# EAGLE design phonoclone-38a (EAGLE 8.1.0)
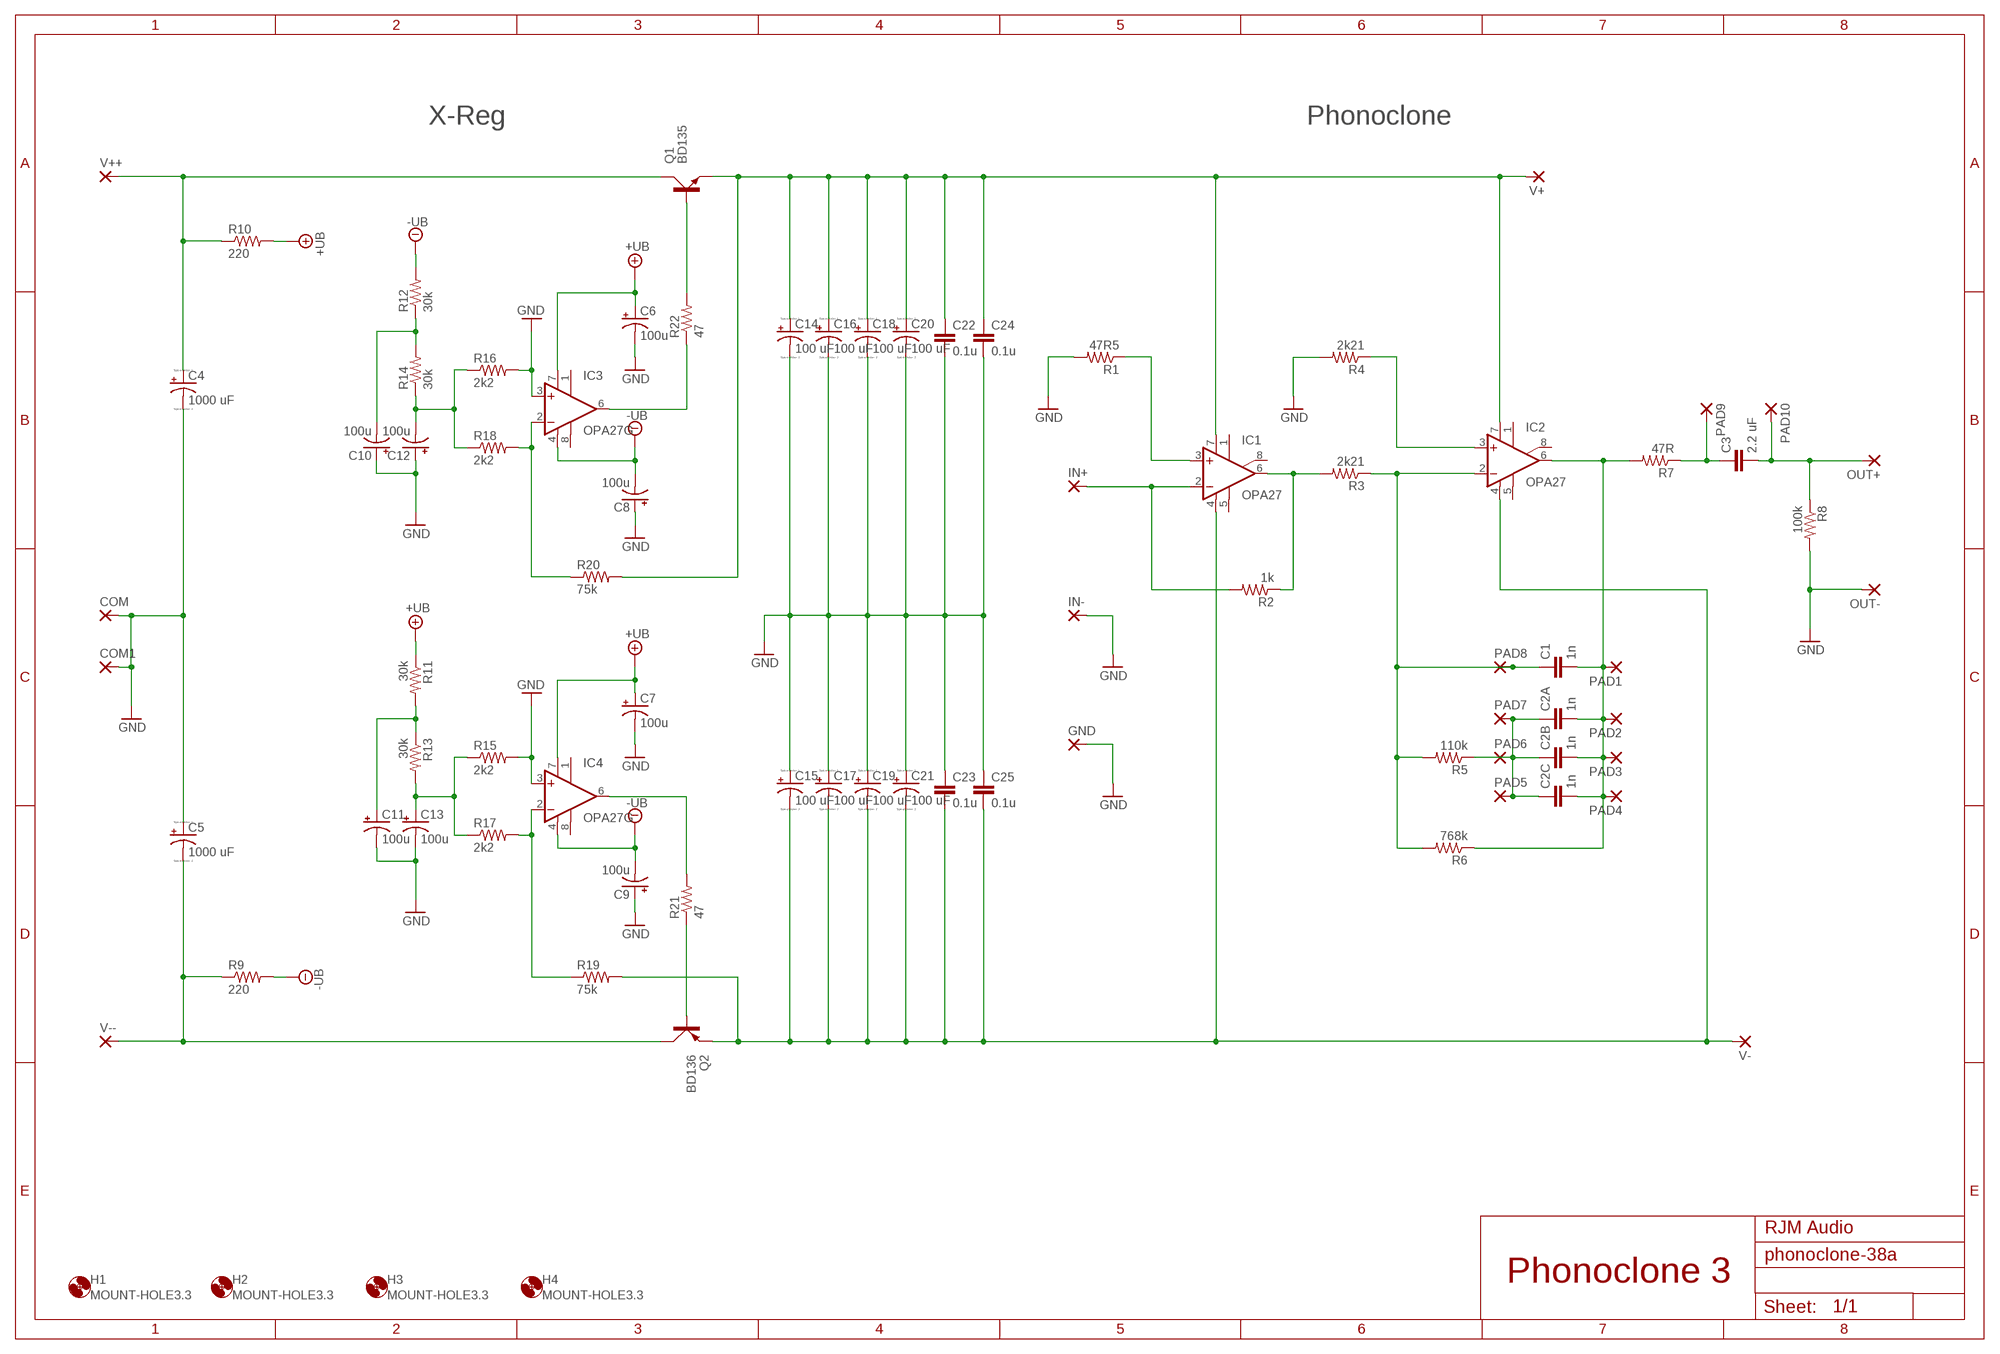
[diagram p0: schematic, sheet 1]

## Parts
C1  1n  C-EU050-045X075  [C050-045X075]
C2A  1n  C-EU050-045X075  [C050-045X075]
C2B  1n  C-EU050-045X075  [C050-045X075]
C2C  1n  C-EU050-045X075  [C050-045X075]
C3  2.2 uF  C-EU375-155X418  [C375-155X418]
C4  1000 uF  CPOL-USE5-10.5  [E5-10,5]
C5  1000 uF  CPOL-USE5-10.5  [E5-10,5]
C6  100u  CPOL-USE2.5-6  [E2,5-6]
C7  100u  CPOL-USE2.5-6  [E2,5-6]
C8  100u  CPOL-USE2.5-6  [E2,5-6]
C9  100u  CPOL-USE2.5-6  [E2,5-6]
C10  100u  CPOL-USE2.5-6  [E2,5-6]
C11  100u  CPOL-USE2.5-6  [E2,5-6]
C12  100u  CPOL-USE2.5-6  [E2,5-6]
C13  100u  CPOL-USE2.5-6  [E2,5-6]
C14  100 uF  CPOL-USE2.5-6  [E2,5-6]
C15  100 uF  CPOL-USE2.5-6  [E2,5-6]
C16  100 uF  CPOL-USE2.5-6  [E2,5-6]
C17  100 uF  CPOL-USE2.5-6  [E2,5-6]
C18  100 uF  CPOL-USE2.5-6  [E2,5-6]
C19  100 uF  CPOL-USE2.5-6  [E2,5-6]
C20  100 uF  CPOL-USE2.5-6  [E2,5-6]
C21  100 uF  CPOL-USE2.5-6  [E2,5-6]
C22  0.1u  C-EU050-024X044  [C050-024X044]
C23  0.1u  C-EU050-024X044  [C050-024X044]
C24  0.1u  C-EU050-024X044  [C050-024X044]
C25  0.1u  C-EU050-024X044  [C050-024X044]
COM  3,17/1,3  [3,17/1,3]
COM1  3,17/1,3  [3,17/1,3]
GND  3,17/1,3  [3,17/1,3]
H1  MOUNT-HOLE3.3  [3,3]
H2  MOUNT-HOLE3.3  [3,3]
H3  MOUNT-HOLE3.3  [3,3]
H4  MOUNT-HOLE3.3  [3,3]
IC1  OPA27  OPA124P  [DIL08]
IC2  OPA27  OPA124P  [DIL08]
IC3  OPA27G  OPA134P  [DIL08]
IC4  OPA27G  OPA134P  [DIL08]
IN+  3,17/1,3  [3,17/1,3]
IN-  3,17/1,3  [3,17/1,3]
OUT+  3,17/1,3  [3,17/1,3]
OUT-  3,17/1,3  [3,17/1,3]
PAD1  2,15/1,0  [2,15/1,0]
PAD2  2,15/1,0  [2,15/1,0]
PAD3  2,15/1,0  [2,15/1,0]
PAD4  2,15/1,0  [2,15/1,0]
PAD5  2,15/1,0  [2,15/1,0]
PAD6  2,15/1,0  [2,15/1,0]
PAD7  2,15/1,0  [2,15/1,0]
PAD8  2,15/1,0  [2,15/1,0]
PAD9  3,17/1,3  [3,17/1,3]
PAD10  3,17/1,3  [3,17/1,3]
Q1  BD135  BD139  [TO126AV]
Q2  BD136  BD140  [TO126AV]
R1  47R5  R-US_0207/10  [0207/10]
R2  1k  R-US_0207/10  [0207/10]
R3  2k21  R-US_0207/10  [0207/10]
R4  2k21  R-US_0207/10  [0207/10]
R5  110k  R-US_0207/10  [0207/10]
R6  768k  R-US_0207/10  [0207/10]
R7  47R  R-US_0207/10  [0207/10]
R8  100k  R-US_0207/10  [0207/10]
R9  220  R-US_0207/10  [0207/10]
R10  220  R-US_0207/10  [0207/10]
R11  30k  R-US_0207/10  [0207/10]
R12  30k  R-US_0207/10  [0207/10]
R13  30k  R-US_0207/10  [0207/10]
R14  30k  R-US_0207/10  [0207/10]
R15  2k2  R-US_0207/10  [0207/10]
R16  2k2  R-US_0207/10  [0207/10]
R17  2k2  R-US_0207/10  [0207/10]
R18  2k2  R-US_0207/10  [0207/10]
R19  75k  R-US_0207/10  [0207/10]
R20  75k  R-US_0207/10  [0207/10]
R21  47  R-US_0207/10  [0207/10]
R22  47  R-US_0207/10  [0207/10]
V+  2,15/1,0  [2,15/1,0]
V++  3,17/1,3  [3,17/1,3]
V-  2,15/1,0  [2,15/1,0]
V--  3,17/1,3  [3,17/1,3]

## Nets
+UB: C6.+ C7.+ IC3.7(V+) IC4.7(V+) R10.2 R11.1
-UB: C8.- C9.- IC3.4(V-) IC4.4(V-) R9.2 R12.2
GND: C4.- C5.+ C6.- C7.- C8.+ C9.+ C10.+ C11.- C12.+ C13.- C14.- C15.+ C16.- C17.+ C18.- C19.+ C20.- C21.+ C22.2 C23.1 C24.2 C25.1 COM1.1(P) COM.1(P) GND.1(P) IC3.3(+IN) IC4.3(+IN) IN-.1(P) OUT-.1(P) R1.2 R4.2 R8.2 R15.2 R16.2
N$1: IC1.6(OUT) R2.1 R3.2
N$2: IC1.3(+IN) R1.1
N$3: IC2.3(+IN) R4.1
N$4: IC3.6(OUT) R22.1
N$5: C2A.1 C2B.1 C2C.1 PAD5.1(P) PAD6.1(P) PAD7.1(P) R5.1
N$6: C1.1 IC2.2(-IN) PAD8.1(P) R3.1 R5.2 R6.2
N$7: Q1.B R22.2
N$8: C11.+ R11.2 R13.1
N$9: IC4.2(-IN) R17.2 R19.1
N$10: Q2.B R21.1
N$11: IC4.6(OUT) R21.2
N$13: IC3.2(-IN) R18.2 R20.1
N$14: C10.- R12.1 R14.2
N$16: C3.1 PAD9.1(P) R7.1
NINV: IC1.2(-IN) IN+.1(P) R2.2
OUT: C1.2 C2A.2 C2B.2 C2C.2 IC2.6(OUT) PAD1.1(P) PAD2.1(P) PAD3.1(P) PAD4.1(P) R6.1 R7.2
OUT+: C3.2 OUT+.1(P) PAD10.1(P) R8.1
V+: C14.+ C16.+ C18.+ C20.+ C22.1 C24.1 IC1.7(V+) IC2.7(V+) Q1.E R20.2 V+.1(P)
V++: C4.+ Q1.C R10.1 V++.1(P)
V-: C15.- C17.- C19.- C21.- C23.2 C25.2 IC1.4(V-) IC2.4(V-) Q2.E R19.2 V-.1(P)
V--: C5.- Q2.C R9.1 V--.1(P)
VREF+: C13.+ R13.2 R15.1 R17.1
VREF-: C12.- R14.1 R16.1 R18.1
Unconnected: IC1.1(TRIM1) IC1.5(TRIM2) IC1.8(SUBS) IC2.1(TRIM1) IC2.5(TRIM2) IC2.8(SUBS) IC3.1(TRIM1) IC3.8(TRIM2) IC4.1(TRIM1) IC4.8(TRIM2)

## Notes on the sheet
- X-Reg | Phonoclone
- RJM Audio
- Phonoclone 3

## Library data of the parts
C1 C2A C2B C2C C3 = resistor:C-EU: CAPACITOR, European symbol
C4 C5 C14-C21 = resistor:CPOL-US: POLARIZED CAPACITOR, American symbol
C6-C13 = rcl:CPOL-US: POLARIZED CAPACITOR, American symbol
C22-C25 = rcl:C-EU: CAPACITOR, European symbol
COM COM1 GND IN+ IN- OUT+ OUT- PAD9 PAD10 V++ V-- = wirepad:3,17/1,3: THROUGH-HOLE PAD
H1-H4 = holes:MOUNT-HOLE: MOUNTING HOLE with drill center marker
IC1 IC2 = burr-brown:OPA124: Difet Operational Amplifier Low Noise, Precision; OC_FARNELL: unknown; OC_NEWARK: unknown
IC3 IC4 = burr-brown:OPA134: Operational Amplifiers SoundPlus(TM) High Performance Audio; MF: TEXAS INSTRUMENTS; MPN: OPA134PA; OC_FARNELL: 1335032; OC_NEWARK: 75C4599
PAD1-PAD8 V+ V- = wirepad:2,15/1,0: THROUGH-HOLE PAD
Q1 = transistor-power:BD139: NPN TRANSISTOR
Q2 = transistor-power:BD140: PNP TRANSISTOR
R1-R8 = resistor:R-US_: RESISTOR, American symbol
R9-R22 = rcl:R-US_: RESISTOR, American symbol

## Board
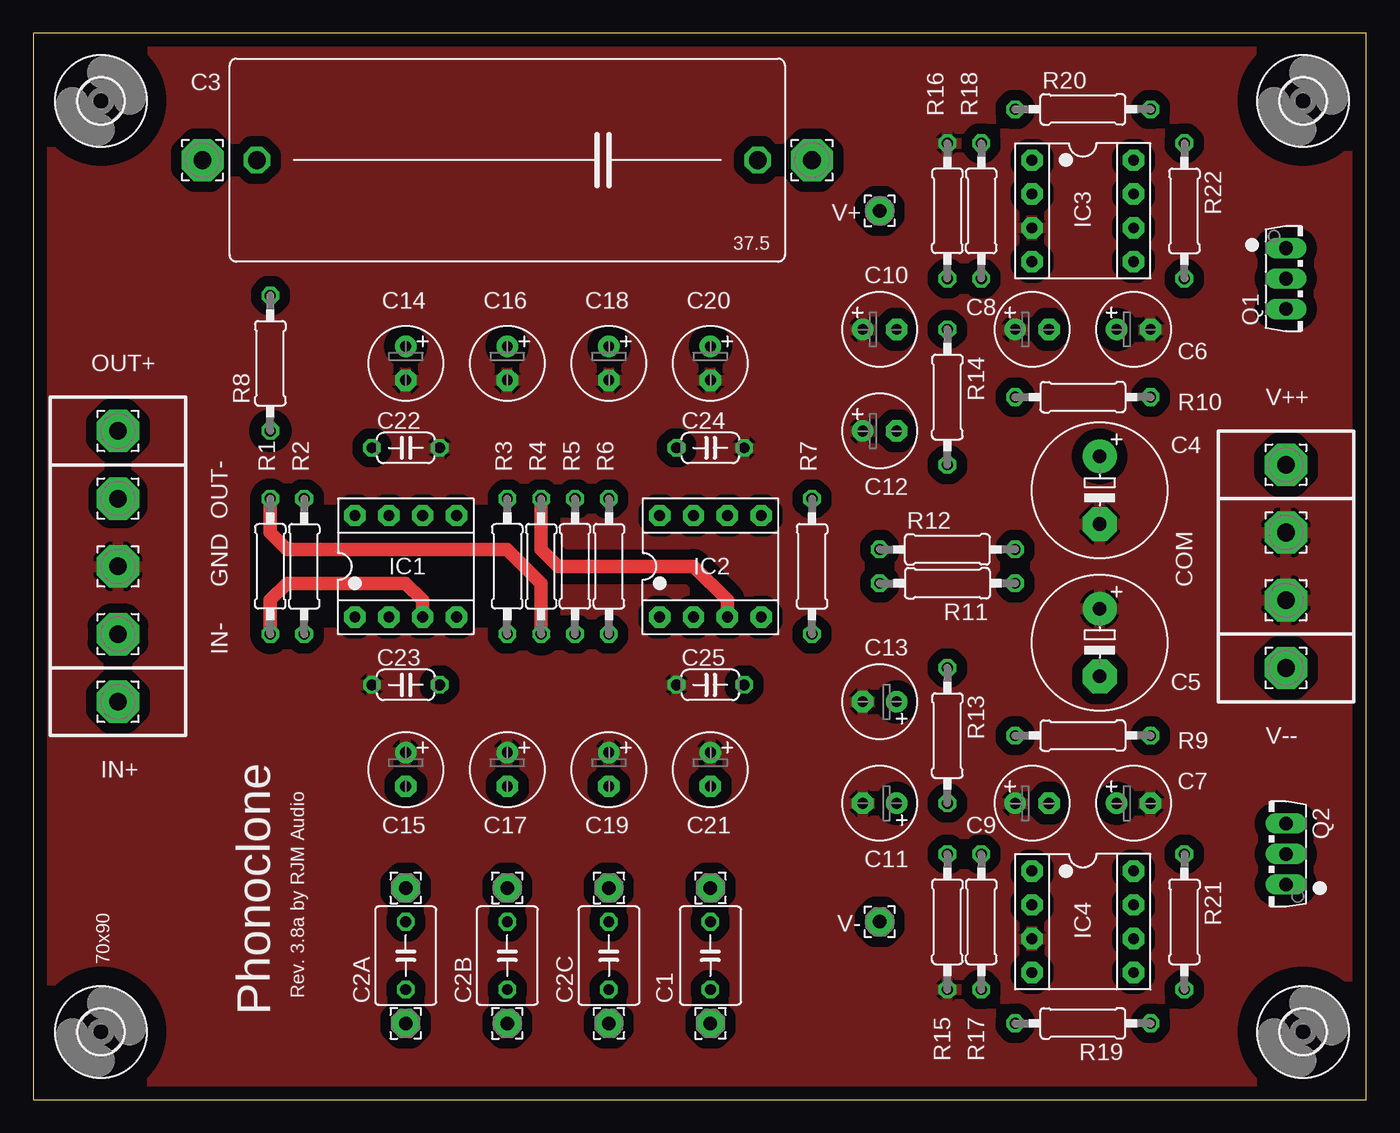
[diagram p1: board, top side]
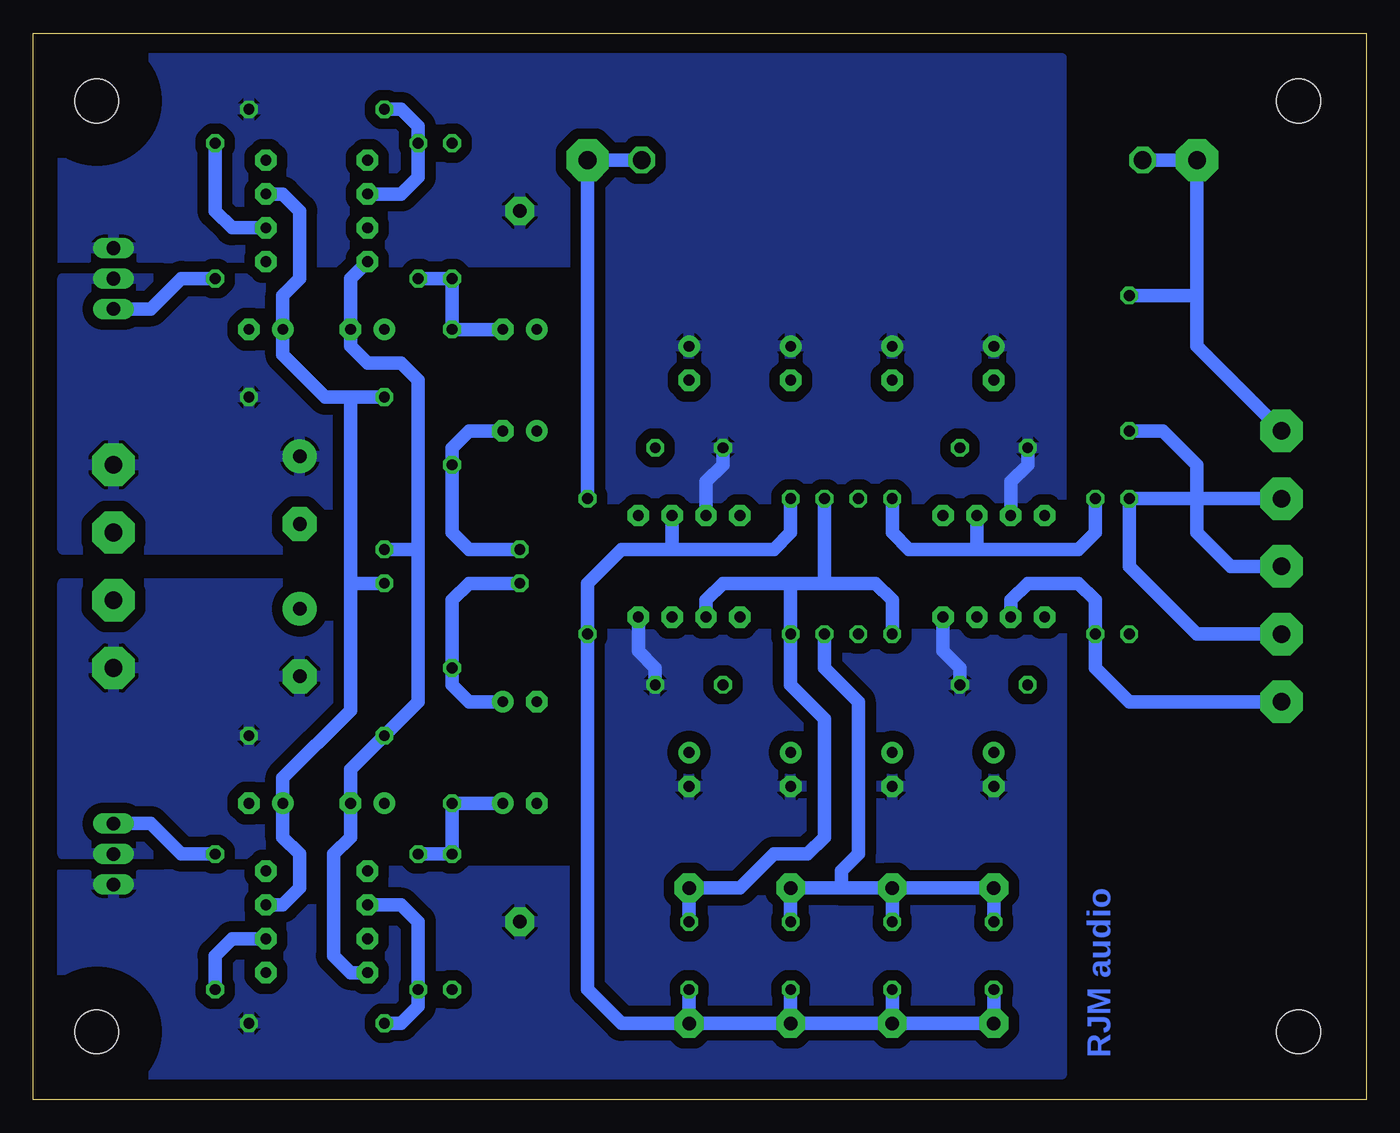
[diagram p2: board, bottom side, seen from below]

Size 100 x 80 mm. Coordinates in mm from the lower left corner, seen from the top.
Outline: 0,0 100,0 100,80 0,80 0,0
Copper layers (1*16): Top 0.035mm / dielectric 1.5mm / Bottom 0.035mm
Design rules "default": minimum track width 10mil, minimum drill 24mil, track to track 8mil, track to pad 8mil, pad to pad 8mil, via to via 8mil, smd to smd 8mil, copper to edge 40mil, drill to drill 8mil, minimum pad ring 10mil, minimum via ring 8mil, stop-mask expansion 4mil, vias tented up to drill 0mil, thermal gap 10mil
tRestrict: area 17.1,49.5 to 18.4,50.8; area 37.5,34.3 to 38.7,35.6; area 18.4,36.2 to 38.7,43.8; 17 lines

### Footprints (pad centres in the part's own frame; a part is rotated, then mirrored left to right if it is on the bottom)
C050-045X075 = drill 0.813 octagon: 1 -2.54,0; 2 2.54,0
C375-155X418 = drill 1.321 octagon: 1 -18.796,0; 2 18.796,0
E5-10,5 = drill 1.016 pad 2.54: + -2.54,0 | drill 1.016 pad 2.54 octagon: - 2.54,0
E2,5-6 = drill 0.813 pad 1.6: + -1.27,0 | drill 0.813 pad 1.6 octagon: - 1.27,0
C050-024X044 = drill 0.813 octagon: 1 -2.54,0; 2 2.54,0
3,17/1,3 = drill 1.321 pad 3.175 octagon: 1 0,0
3,3 = hole 3.3: 0,0
DIL08 = drill 0.813 pad 1.6 octagon: 1 -3.81,-3.81; 2 -1.27,-3.81; 3 1.27,-3.81; 4 3.81,-3.81; 5 3.81,3.81; 6 1.27,3.81; 7 -1.27,3.81; 8 -3.81,3.81
2,15/1,0 = drill 1.016 pad 2.159 octagon: 1 0,0
TO126AV = drill 1.016 long: B 2.286,-1.27; C 0,-1.27; E -2.286,-1.27
0207/10 = drill 0.813 octagon: 1 -5.08,0; 2 5.08,0

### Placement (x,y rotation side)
C1  50.8,10.79 270 top
C2A  27.94,10.79 270 top
C2B  35.56,10.79 270 top
C2C  43.18,10.79 270 top
C3  35.56,70.48 180 top
C4  80.01,45.72 270 top
C5  80.01,34.29 270 top
C6  82.55,57.79 0 top
C7  82.55,22.22 0 top
C8  74.93,57.79 0 top
C9  74.93,22.22 0 top
C10  63.5,50.16 0 top
C11  63.5,29.84 180 top
C12  63.5,57.79 0 top
C13  63.5,22.22 180 top
C14  27.94,55.25 270 top
C15  27.94,24.76 270 top
C16  35.56,55.25 270 top
C17  35.56,24.76 270 top
C18  43.18,55.25 270 top
C19  43.18,24.76 270 top
C20  50.8,55.25 270 top
C21  50.8,24.76 270 top
C22  27.94,48.9 0 top
C23  27.94,31.11 0 top
C24  50.8,48.9 0 top
C25  50.8,31.11 0 top
COM  93.98,37.47 0 top
COM1  93.98,42.55 0 top
GND  6.35,40.01 0 top
H1  5.08,74.93 0 top
H2  95.25,74.93 0 top
H3  5.08,5.08 0 top
H4  95.25,5.08 0 top
IC1  27.94,40.01 0 top
IC2  50.8,40.01 0 top
IC3  78.74,66.67 270 top
IC4  78.74,13.34 270 top
IN+  6.35,29.84 0 top
IN-  6.35,34.93 0 top
OUT+  6.35,50.16 0 top
OUT-  6.35,45.09 0 top
PAD1  27.94,5.71 0 top
PAD2  35.56,5.71 0 top
PAD3  43.18,5.71 0 top
PAD4  50.8,5.71 0 top
PAD5  35.56,15.88 0 top
PAD6  43.18,15.88 0 top
PAD7  27.94,15.88 0 top
PAD8  50.8,15.88 0 top
PAD9  58.42,70.48 0 top
PAD10  12.7,70.48 0 top
Q1  95.25,61.59 270 top
Q2  92.71,18.41 90 top
R1  17.78,40.01 90 top
R2  20.32,40.01 270 top
R3  35.56,40.01 90 top
R4  38.1,40.01 270 top
R5  40.64,40.01 90 top
R6  43.18,40.01 270 top
R7  58.42,40.01 270 top
R8  17.78,55.25 270 top
R9  78.74,27.3 180 top
R10  78.74,52.71 180 top
R11  68.58,38.73 180 top
R12  68.58,41.27 0 top
R13  68.58,27.3 270 top
R14  68.58,52.71 270 top
R15  68.58,13.34 270 top
R16  68.58,66.67 90 top
R17  71.12,13.34 270 top
R18  71.12,66.67 90 top
R19  78.74,5.71 0 top
R20  78.74,74.3 0 top
R21  86.36,13.34 270 top
R22  86.36,66.67 270 top
V+  63.5,66.67 0 top
V++  93.98,47.62 0 top
V-  63.5,13.34 180 top
V--  93.98,32.39 0 top

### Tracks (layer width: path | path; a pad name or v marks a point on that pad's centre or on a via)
+UB
  Bottom 1.016: IC3.7 81.28,67.94 80.01,66.67 80.01,61.59 81.28,60.33 C6.+ 81.28,55.88 78.11,52.71 76.2,52.71 | 76.2,38.73 76.2,52.71 | 76.2,52.71 R10.2 | R11.1 76.2,38.73 | 76.2,38.73 76.2,29.21 81.28,24.13 C7.+ 81.28,19.68 80.01,18.41 80.01,15.88 81.28,14.61 IC4.7
-UB
  Bottom 1.016: IC3.4 76.2,61.59 C8.- 76.2,56.52 74.93,55.25 72.39,55.25 71.12,53.98 71.12,41.27 | IC4.4 76.2,9.53 77.47,10.79 77.47,18.41 76.2,19.68 C9.- 76.2,24.76 R9.2 71.12,29.84 71.12,41.27 | R12.2 71.12,41.27
GND
  Top 1.016: R1.2 17.78,42.55 19.05,41.27 35.56,41.27 38.1,38.73 R4.2
  Bottom 1.016: 12.7,45.09 12.7,47.62 15.24,50.16 R8.2 | IN-.1 12.7,34.93 17.78,40.01 R1.2 12.7,45.09 | 12.7,45.09 OUT-.1 | GND.1 10.16,40.01 12.7,42.55 12.7,45.09
  pour Top (isolate 0.813): -1.27,81.28 101.6,81.28 101.6,-1.91 -1.27,-1.91
N$1
  Bottom 1.016: R2.1 20.32,42.55 21.59,41.27 29.21,41.27 | R3.2 35.56,42.55 34.29,41.27 29.21,41.27 | 29.21,41.27 IC1.6
N$2
  Top 1.016: IC1.3 29.21,37.47 27.94,38.73 19.05,38.73 17.78,37.47 R1.1
N$3
  Top 1.016: R4.1 38.1,41.27 39.37,40.01 49.53,40.01 52.07,37.47 IC2.3
N$4
  Bottom 1.016: IC3.6 85.09,65.41 86.36,66.67 R22.1
N$5
  Bottom 1.016: C2C.1 PAD6.1 39.37,15.88 | C2B.1 PAD5.1 | C2A.1 PAD7.1 PAD5.1 | R5.1 40.64,32.39 38.1,29.84 38.1,18.41 39.37,17.14 39.37,15.88 | 39.37,15.88 PAD5.1
N$6
  Bottom 1.016: C1.1 PAD8.1 46.99,15.88 44.45,18.41 41.91,18.41 40.64,19.68 40.64,28.57 43.18,31.11 R6.2 43.18,38.73 | R3.1 35.56,37.47 36.83,38.73 40.64,38.73 | IC2.2 49.53,37.47 48.26,38.73 43.18,38.73 | 43.18,38.73 40.64,38.73 | 40.64,38.73 R5.2
N$7
  Bottom 1.016: Q1.B 91.19,59.31 88.9,61.59 R22.2
N$8
  Bottom 1.016: R11.2 67.31,38.73 68.58,37.47 R13.1 68.58,31.11 67.31,29.84 C11.+
N$9
  Bottom 1.016: IC4.2 72.39,14.61 71.12,13.34 R17.2 71.12,6.99 72.39,5.71 R19.1
N$10
  Bottom 1.016: Q2.B 91.19,20.7 88.9,18.41 R21.1
N$11
  Bottom 1.016: IC4.6 85.09,12.06 86.36,10.79 R21.2
N$13
  Bottom 1.016: IC3.2 72.39,67.94 71.12,69.21 R18.2 71.12,73.02 72.39,74.3 R20.1
N$14
  Bottom 1.016: C10.- 67.31,50.16 68.58,48.9 R14.2 68.58,42.55 67.31,41.27 R12.1
N$16
  Bottom 1.016: R7.1 PAD9.1 C3.1
NINV
  Bottom 1.016: IC1.2 26.67,37.47 25.4,38.73 21.59,38.73 20.32,37.47 R2.2 20.32,32.39 17.78,29.84 IN+.1
OUT
  Bottom 1.016: C2C.2 PAD3.1 | C2B.2 PAD2.1 | C2A.2 PAD1.1 PAD2.1 | R6.1 43.18,42.55 44.45,41.27 52.07,41.27 | 52.07,41.27 55.88,41.27 58.42,38.73 R7.2 58.42,8.26 55.88,5.71 PAD4.1 | IC2.6 52.07,41.27 | C1.2 PAD4.1 | PAD2.1 PAD3.1 | PAD3.1 PAD4.1
OUT+
  Bottom 1.016: OUT+.1 12.7,56.52 12.7,60.33 | C3.2 PAD10.1 12.7,60.33 | R8.1 12.7,60.33
V+
  Bottom 1.016: IC2.7 49.53,46.36 48.26,47.62 C24.1 | IC1.7 26.67,46.36 25.4,47.62 C22.1
  pour Bottom (isolate 0.813, rank 3): 22.86,45.09 22.86,78.1 97.79,78.1 97.79,62.87 58.42,62.87 58.42,45.09
V++
  pour Bottom (isolate 0.813): 97.79,41.27 97.79,61.59 76.2,61.59 76.2,41.27
V-
  Bottom 1.016: IC1.4 31.75,33.66 30.48,32.39 C23.2 | IC2.4 54.61,33.66 53.34,32.39 C25.2
  pour Bottom (isolate 0.813, rank 3): 22.86,34.93 22.86,1.91 97.79,1.91 97.79,17.14 58.42,17.14 58.42,34.93
V--
  pour Bottom (isolate 0.813): 76.2,38.73 76.2,18.41 97.79,18.41 97.79,38.73
VREF+
  Bottom 1.016: R17.1 R15.1 R13.2 C13.+
VREF-
  Bottom 1.016: R18.1 R16.1 R14.1 C12.-

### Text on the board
Bottom: RJM audio
tPlace: 37.5 | 70x90 | Rev. 3.8a by RJM Audio | Phonoclone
